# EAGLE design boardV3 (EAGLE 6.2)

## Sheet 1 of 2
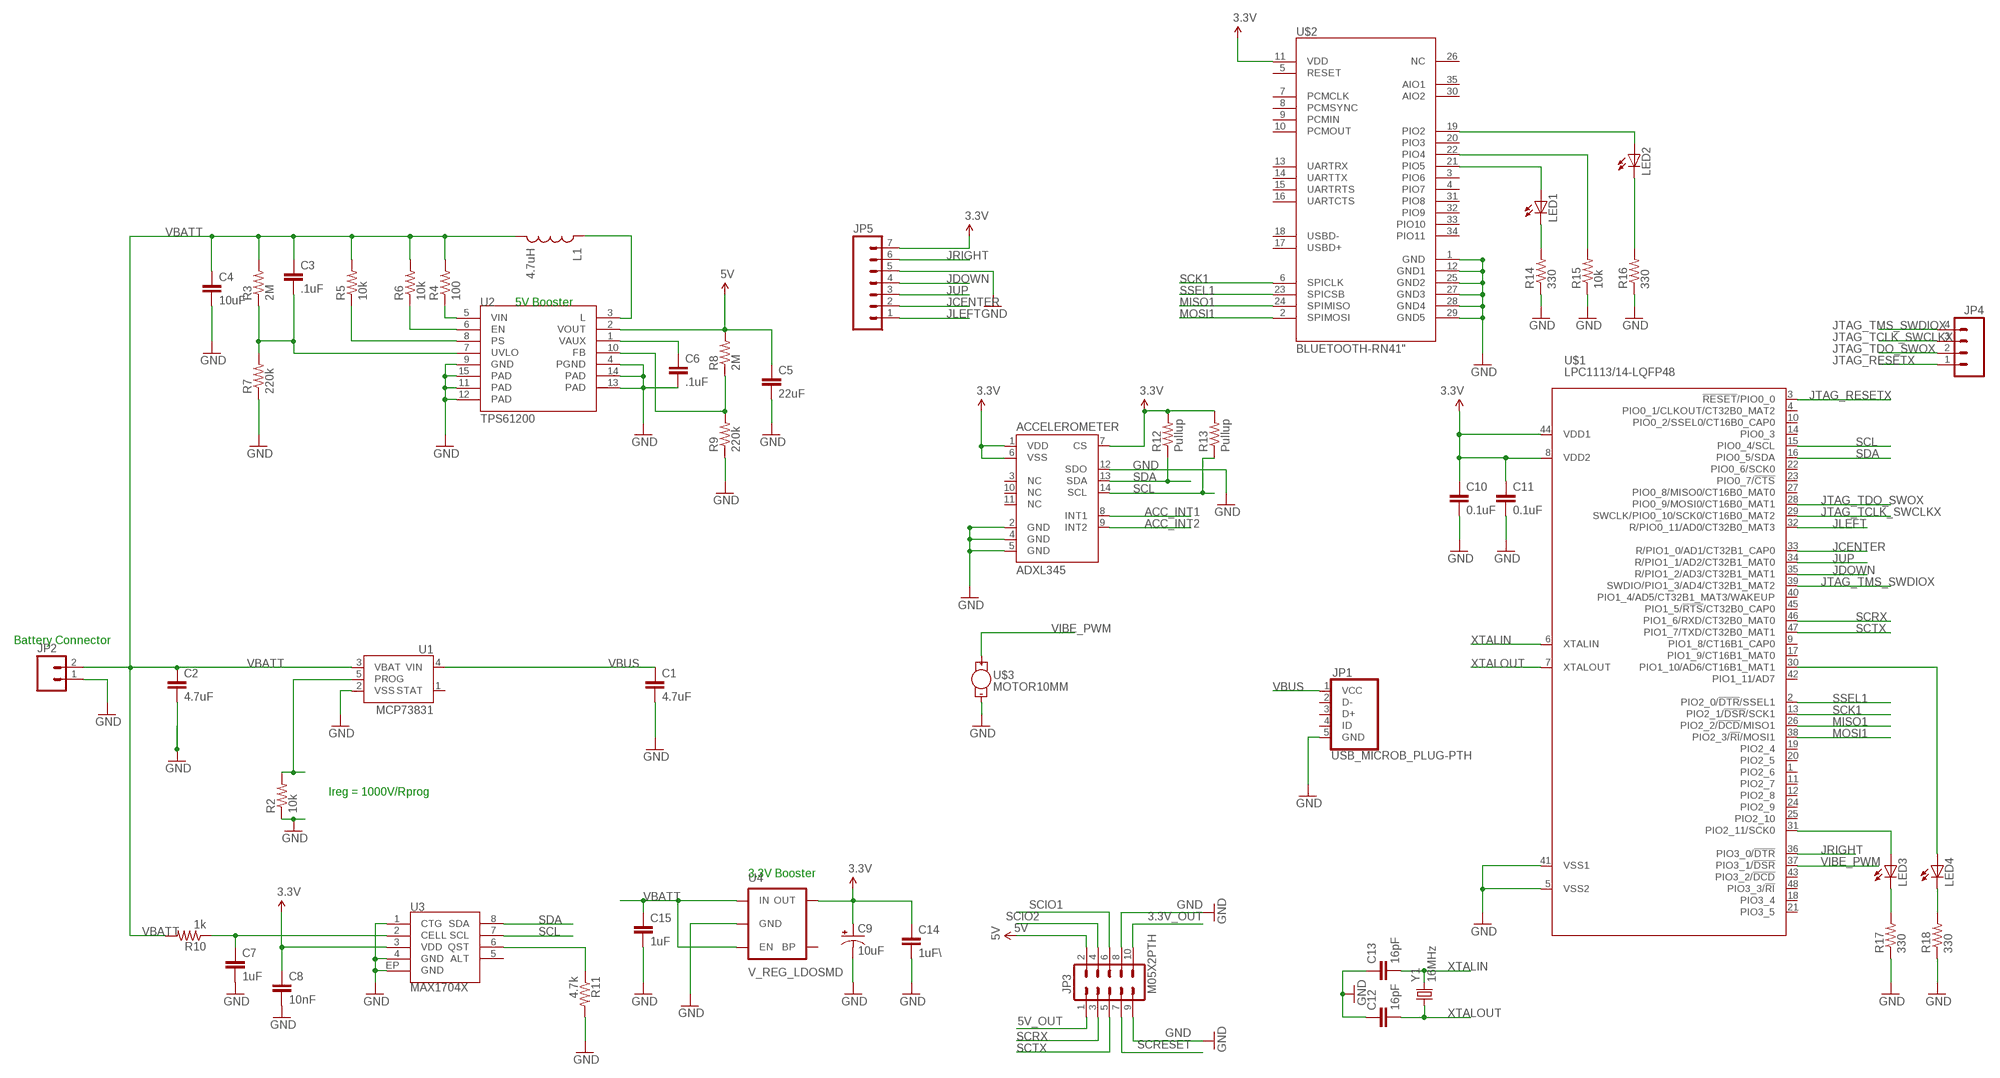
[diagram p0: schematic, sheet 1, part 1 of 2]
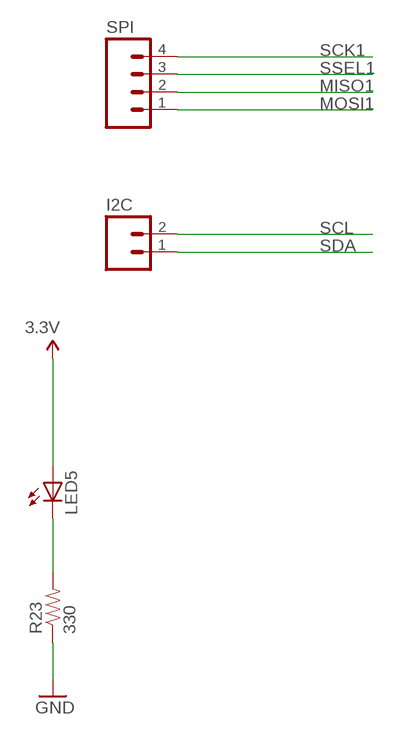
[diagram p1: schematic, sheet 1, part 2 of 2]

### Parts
ACCELEROMETER  ADXL345  [LGA14]
C1  4.7uF  CAP0603-CAP  [0603-CAP]
C2  4.7uF  CAP0603-CAP  [0603-CAP]
C3  .1uF  CAP0603-CAP  [0603-CAP]
C4  10uF  CAP0603-CAP  [0603-CAP]
C5  22uF  CAP0603-CAP  [0603-CAP]
C6  .1uF  CAP0603-CAP  [0603-CAP]
C7  1uF  CAP0603-CAP  [0603-CAP]
C8  10nF  CAP0603-CAP  [0603-CAP]
C9  10uF  10UF-TANT  [EIA3216]
C10  0.1uF  CAP0603-CAP  [0603-CAP]
C11  0.1uF  CAP0603-CAP  [0603-CAP]
C12  16pF  CAP0603-CAP  [0603-CAP]
C13  16pF  CAP0603-CAP  [0603-CAP]
C14  1uF\  CAP0603-CAP  [0603-CAP]
C15  1uF  CAP0603-CAP  [0603-CAP]
I2C  M02POGO_PIN_HOLES_ONLY  [1X02_PP_HOLES_ONLY]
JP1  USB_MICROB_PLUG-PTH  [MICRO-B-RA-TH]
JP2  M02-JST-2-PTH-NO_SILK  [JST-2-PTH-NS]
JP3  M05X2PTH  [AVR_ICSP]
JP4  M04POLAR  [MOLEX-1X4]
JP5  M07  [1X07]
L1  4.7uH  INDUCTOR.  [CDRH2D09]
LED1  LED0603  [LED-0603]
LED2  LED0603  [LED-0603]
LED3  LED0603  [LED-0603]
LED4  LED0603  [LED-0603]
LED5  LED0603  [LED-0603]
R2  10k  RESISTOR0603-RES  [0603-RES]
R3  2M  RESISTOR0603-RES  [0603-RES]
R4  100  RESISTOR0603-RES  [0603-RES]
R5  10k  RESISTOR0603-RES  [0603-RES]
R6  10k  RESISTOR0603-RES  [0603-RES]
R7  220k  RESISTOR0603-RES  [0603-RES]
R8  2M  RESISTOR0603-RES  [0603-RES]
R9  220k  RESISTOR0603-RES  [0603-RES]
R10  1k  RESISTOR0603-RES  [0603-RES]
R11  4.7k  RESISTOR0603-RES  [0603-RES]
R12  Pullup  RESISTOR0402-RES  [0402-RES]
R13  Pullup  RESISTOR0402-RES  [0402-RES]
R14  330  RESISTOR0603-RES  [0603-RES]
R15  10k  RESISTOR0603-RES  [0603-RES]
R16  330  RESISTOR0603-RES  [0603-RES]
R17  330  RESISTOR0603-RES  [0603-RES]
R18  330  RESISTOR0603-RES  [0603-RES]
R23  330  RESISTOR0603-RES  [0603-RES]
SPI  M04POLAR  [MOLEX-1X4]
U1  MCP73831  [SOT23-5]
U2  TPS61200  [QFN-10_PAD]
U3  MAX1704X  [TDFN-8]
U4  V_REG_LDOSMD  [SOT23-5]
U$1  LPC1113/14-LQFP48  [LQFP48]
U$2  BLUETOOTH-RN41"  [RN41]
U$3  MOTOR10MM  [VIBE-MOTOR-10MM]
Y1  16MHz  CRYSTAL5X3  [CRYSTAL-SMD-5X3]

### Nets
3.3V: ACCELEROMETER.1(VDD) ACCELEROMETER.6(VSS) ACCELEROMETER.7(CS) C8.1 C9.A(+) C10.1 C11.1 C14.1 JP5.7 LED5.A R12.2 R13.2 U3.3(VDD) U4.5(OUT) U$1.8(VDD2) U$1.44(VDD1) U$2.11(VDD) ; also sheet 2
3.3V_OUT: JP3.10
5V: C5.1 JP3.2 R8.2 U2.2(VOUT)
5V_OUT: JP3.1
ACC_INT1: ACCELEROMETER.8(INT1)
ACC_INT2: ACCELEROMETER.9(INT2)
GND: ACCELEROMETER.2(GND) ACCELEROMETER.4(GND) ACCELEROMETER.5(GND) ACCELEROMETER.12(SDO) C1.2 C2.2 C4.2 C5.2 C6.2 C7.2 C8.2 C9.C(-) C10.2 C11.2 C12.1 C13.1 C14.2 C15.2 JP1.5(GND) JP2.1 JP3.8 JP3.9 JP5.5 R2.1 R7.1 R9.1 R11.2 R14.1 R15.1 R16.1 R17.1 R18.1 R23.1 U1.2(VSS) U2.4(PGND) U2.9(GND) U2.11(PAD) U2.12(PAD) U2.13(PAD) U2.14(PAD) U2.15(PAD) U3.1(CTG) U3.4(GND) U3.EP(GND) U4.2(GND) U$1.5(VSS2) U$1.41(VSS1) U$2.1(GND) U$2.12(GND1) U$2.25(GND2) U$2.27(GND3) U$2.28(GND4) U$2.29(GND5) U$3.- ; also sheet 2
JCENTER: JP5.2 U$1.33(R/PIO1_0/AD1/CT32B1_CAP0) ; also sheet 2
JDOWN: JP5.4 U$1.35(R/PIO1_2/AD3/CT32B1_MAT1) ; also sheet 2
JLEFT: JP5.1 U$1.32(R/PIO0_11/AD0/CT32B0_MAT3) ; also sheet 2
JRIGHT: JP5.6 U$1.36(PIO3_0/!DTR!) ; also sheet 2
JTAG_RESETX: JP4.1 U$1.3(!RESET!/PIO0_0)
JTAG_TCLK_SWCLKX: JP4.3 U$1.29(SWCLK/PIO0_10/SCK0/CT16B0_MAT2)
JTAG_TDO_SWOX: JP4.2 U$1.28(PIO0_9/MOSI0/CT16B0_MAT1)
JTAG_TMS_SWDIOX: JP4.4 U$1.39(SWDIO/PIO1_3/AD4/CT32B1_MAT2)
JUP: JP5.3 U$1.34(R/PIO1_1/AD2/CT32B1_MAT0) ; also sheet 2
MISO1: SPI.2 U$1.26(PIO2_2/!DCD!/MISO1) U$2.24(SPIMISO)
MOSI1: SPI.1 U$1.38(PIO2_3/!RI!/MOSI1) U$2.2(SPIMOSI)
N$1: LED2.A U$2.19(PIO2)
N$2: R2.2 U1.5(PROG)
N$3: C3.2 R3.1 R7.2 U2.7(UVLO)
N$4: C6.1 U2.1(VAUX)
N$5: R6.1 U2.6(EN)
N$6: R5.1 U2.8(PS)
N$7: L1.P$1 U2.3(L)
N$8: R8.1 R9.2 U2.10(FB)
N$9: C7.1 R10.1 U3.2(CELL)
N$10: R11.1 U3.6(QST)
N$11: R15.2 U$2.22(PIO4)
N$12: LED1.A U$2.21(PIO5)
N$13: LED1.C R14.2
N$14: LED2.C R16.2
N$15: LED3.A U$1.31(PIO2_11/SCK0)
N$16: LED4.A U$1.30(PIO1_10/AD6/CT16B1_MAT1)
N$17: LED3.C R17.2
N$18: LED4.C R18.2
N$21: LED5.C R23.2
SCIO1: JP3.6
SCIO2: JP3.4
SCK1: SPI.4 U$1.13(PIO2_1/!DSR!/SCK1) U$2.6(SPICLK)
SCL: ACCELEROMETER.14(SCL) I2C.2 R13.1 U3.7(SCL) U$1.15(PIO0_4/SCL)
SCRESET: JP3.7
SCRX: JP3.3 U$1.46(PIO1_6/RXD/CT32B0_MAT0)
SCTX: JP3.5 U$1.47(PIO1_7/TXD/CT32B0_MAT1)
SDA: ACCELEROMETER.13(SDA) I2C.1 R12.1 U3.8(SDA) U$1.16(PIO0_5/SDA)
SSEL1: SPI.3 U$1.2(PIO2_0/!DTR!/SSEL1) U$2.23(SPICSB)
VBATT: C2.1 C3.1 C4.1 C15.1 JP2.2 L1.P$2 R3.2 R4.2 R5.2 R6.2 R10.2 U1.3(VBAT) U4.1(IN) U4.3(EN)
VBUS: C1.1 JP1.1(VCC) U1.4(VIN)
VIBE_PWM: U$1.37(PIO3_1/!DSR!) U$3.+
VIN: R4.1 U2.5(VIN)
XTALIN: C13.2 U$1.6(XTALIN) Y1.3
XTALOUT: C12.2 U$1.7(XTALOUT) Y1.1
Unconnected: ACCELEROMETER.3(NC) ACCELEROMETER.10(NC) ACCELEROMETER.11(NC) JP1.2(D-) JP1.3(D+) JP1.4(ID) U1.1(STAT) U3.5(ALT) U4.4(BP) U$1.1(PIO2_6) U$1.4(PIO0_1/CLKOUT/CT32B0_MAT2) U$1.9(PIO1_8/CT16B1_CAP0) U$1.10(PIO0_2/SSEL0/CT16B0_CAP0) U$1.11(PIO2_7) U$1.12(PIO2_8) U$1.14(PIO0_3) U$1.17(PIO1_9/CT16B1_MAT0) U$1.18(PIO3_4) U$1.19(PIO2_4) U$1.20(PIO2_5) U$1.21(PIO3_5) U$1.22(PIO0_6/SCK0) U$1.23(PIO0_7/!CTS!) U$1.24(PIO2_9) U$1.25(PIO2_10) U$1.27(PIO0_8/MISO0/CT16B0_MAT0) U$1.40(PIO1_4/AD5/CT32B1_MAT3/WAKEUP) U$1.42(PIO1_11/AD7) U$1.43(PIO3_2/!DCD!) U$1.45(PIO1_5/!RTS!/CT32B0_CAP0) U$1.48(PIO3_3/!RI!) U$2.3(PIO6) U$2.4(PIO7) U$2.5(RESET) U$2.7(PCMCLK) U$2.8(PCMSYNC) U$2.9(PCMIN) U$2.10(PCMOUT) U$2.13(UARTRX) U$2.14(UARTTX) U$2.15(UARTRTS) U$2.16(UARTCTS) U$2.17(USBD+) U$2.18(USBD-) U$2.20(PIO3) U$2.26(NC) U$2.30(AIO2) U$2.31(PIO8) U$2.32(PIO9) U$2.33(PIO10) U$2.34(PIO11) U$2.35(AIO1)

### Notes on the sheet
- 5V Booster
- Battery Connector
- Ireg = 1000V/Rprog
- 3.3V Booster

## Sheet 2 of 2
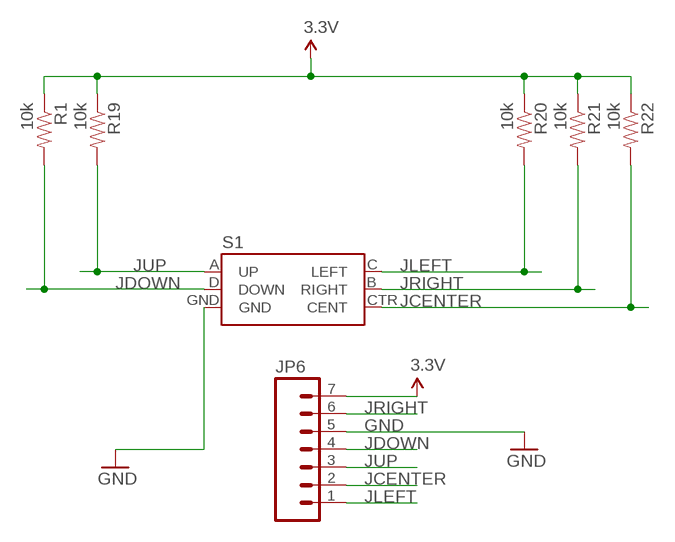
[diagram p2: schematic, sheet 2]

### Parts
JP6  M07  [1X07]
R1  10k  RESISTOR0603-RES  [0603-RES]
R19  10k  RESISTOR0603-RES  [0603-RES]
R20  10k  RESISTOR0603-RES  [0603-RES]
R21  10k  RESISTOR0603-RES  [0603-RES]
R22  10k  RESISTOR0603-RES  [0603-RES]
S1  JOYSTICK_MINI  [JOYSTICK_MINI]

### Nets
3.3V: JP6.7 R1.1 R19.1 R20.1 R21.1 R22.1 ; also sheet 1
GND: JP6.5 S1.GND ; also sheet 1
JCENTER: JP6.2 R22.2 S1.CTR(CENT) ; also sheet 1
JDOWN: JP6.4 R1.2 S1.D(DOWN) ; also sheet 1
JLEFT: JP6.1 R20.2 S1.C(LEFT) ; also sheet 1
JRIGHT: JP6.6 R21.2 S1.B(RIGHT) ; also sheet 1
JUP: JP6.3 R19.2 S1.A(UP) ; also sheet 1

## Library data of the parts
ACCELEROMETER = SparkFun-Sensors:ADXL345: 3-axis SPI/I2C 2/4/8/16g accelerometer
C1-C8 C10-C15 = SparkFun-Passives:CAP: Capacitor
C9 = SparkFun-Capacitors:10UF-TANT: 10uF Tantalum SMT; PROD_ID: CAP-00811
I2C JP2 = SparkFun-Connectors:M02: Header 2
JP1 = SparkFun-Connectors:USB_MICROB_PLUG: USB Micro-B Plug Comes in a variety of packages. Check out Hirose's ZX-x0 line: http://www.hirose.co.jp/cataloge_hp/e24200011.pdf
JP3 = SparkFun-Connectors:M05X2: Header 5x2 Standard 10-pin dual row 0.1" header. Commonly used with AVR-ISP. Use with Spark Fun Electronics SKU: PRT-00778
JP4 SPI = SparkFun-Connectors:M04: Header 4 Standard 4-pin 0.1" header. Use with straight break away headers (SKU : PRT-00116), right angle break away headers (PRT-00553), swiss pins (PRT-00743), machine pins (PRT-00117), and female headers (PRT-00115). Molex polarized connector foot print use with SKU : PRT-08231 with associated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
JP5 JP6 = SparkFun-Connectors:M07: Header 7 Standard 7-pin 0.1" header. Use with straight break away headers (SKU : PRT-00116), right angle break away headers (PRT-00553), swiss pins (PRT-00743), machine pins (PRT-00117), and female headers (PRT-00115). NOTES ON THE VARIANTS LOCK and LOCK_LONGPADS... This footprint was designed to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
L1 = SparkFun-Passives:INDUCTOR: Inductors
LED1-LED5 = SparkFun-LED:LED: LEDs
R1 R8 R9 R19-R22 = SparkFun-Resistors:RESISTOR: Resistor
R2-R7 R10-R18 R23 = SparkFun-Passives:RESISTOR: Resistor
S1 = SparkFun-Electromechanical:JOYSTICK_MINI: Small 5-way tactile joystick, COM-10063 4UCON SF303GJ26
U1 = SparkFun-PowerIC:MCP73831: Miniature single cell, fully integrated Li-Ion, Li-polymer charge management controller http://ww1.microchip.com/downloads/en/DeviceDoc/21984a.pdf IC-09995; PROD_ID: IC-09995
U2 = SparkFun-PowerIC:TPS61200: DC to DC Booster IC-10035; PROD_ID: IC-10035
U3 = SparkFun-PowerIC:MAX1704X: MAX17043/MAX17044: Battery Fuel Guage (43 is 1cell, 44 is 2cell)
U4 = SparkFun-PowerIC:V_REG_LDO: Voltage Regulator LDO Standard 150mA LDO voltage regulator in SOT-23 layout. Micrel part MIC5205. BP (by-pass) pin is used to lower output noise with 470pF cap.
U$1 = lpc1100v1.1:LPC1113/14-LQFP48: NXP Semiconductors LPC11xx microcontrollers ARM 32-bit Cortex-M0 Microcontroller with MPU CPU clock up to 50MHz Up to 32KByte on-chip Flash ROM with In-System Programming (ISP) and In-Application Programming (IAP) via On-Chip Bootloader Up to 8KByte SRAM Nested Vectored Interrupt Controller Up to 2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
U$2 = SparkFun-RF:BLUETOOTH-RN41: Bluetooth SMD module
U$3 = SparkFun-Electromechanical:MOTOR: Vibration Motor- ROB-08449
Y1 = SparkFun-FreqCtrl:CRYSTAL: Various standard crystals. Proven footprints. Spark Fun Electronics SKU : COM-00534

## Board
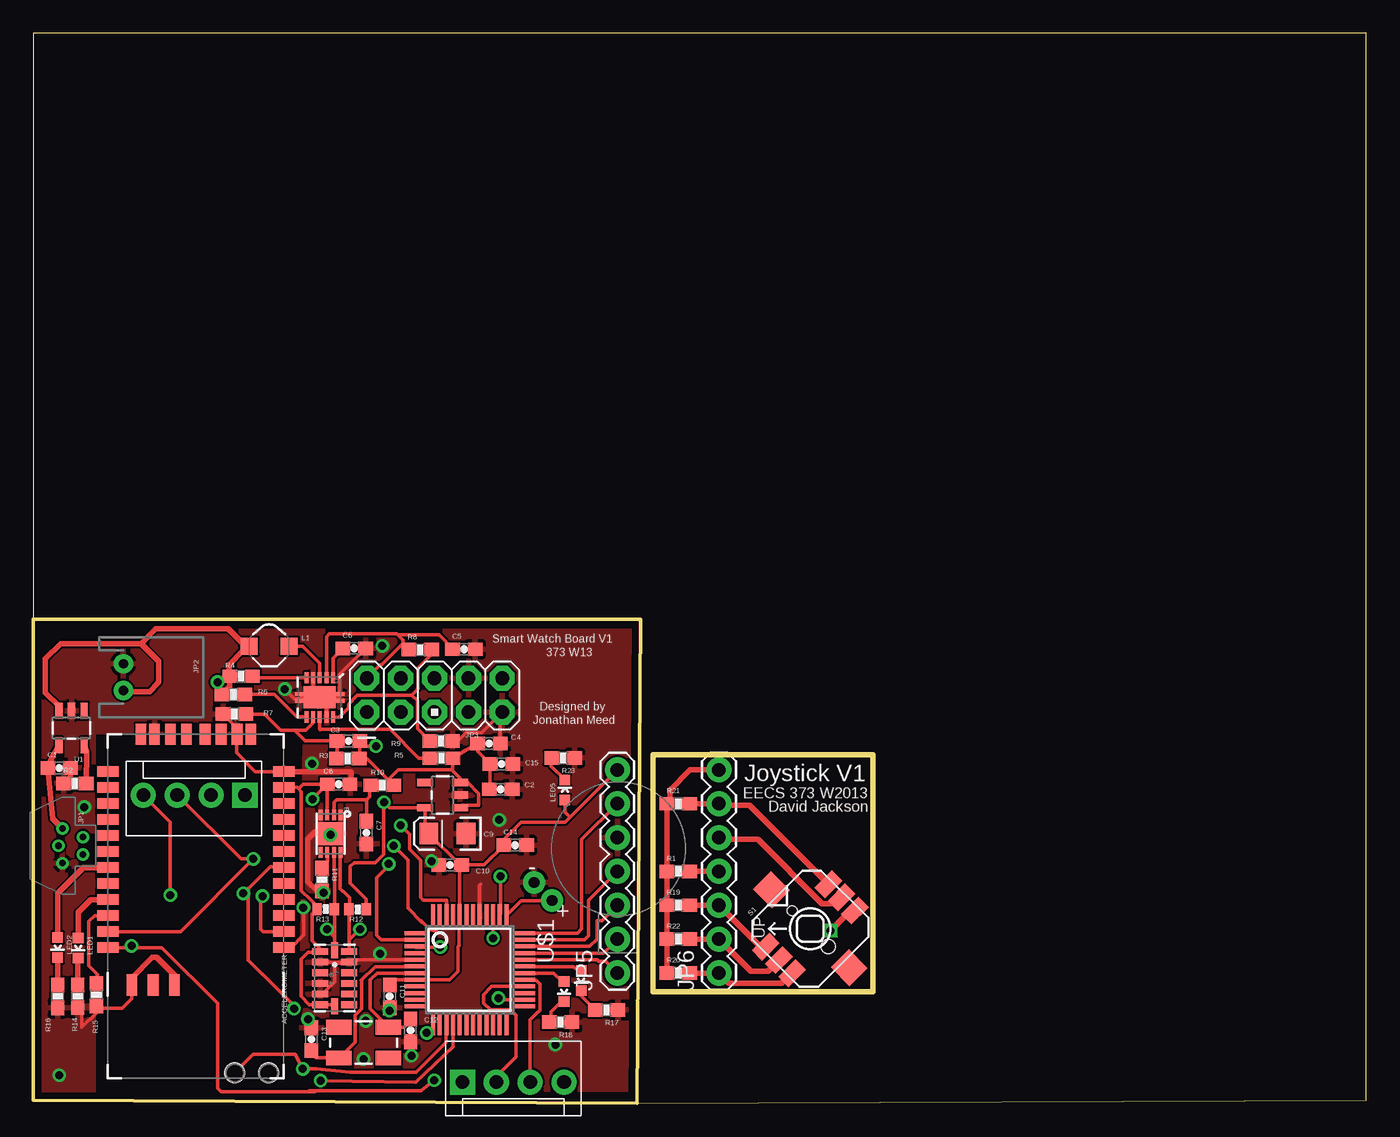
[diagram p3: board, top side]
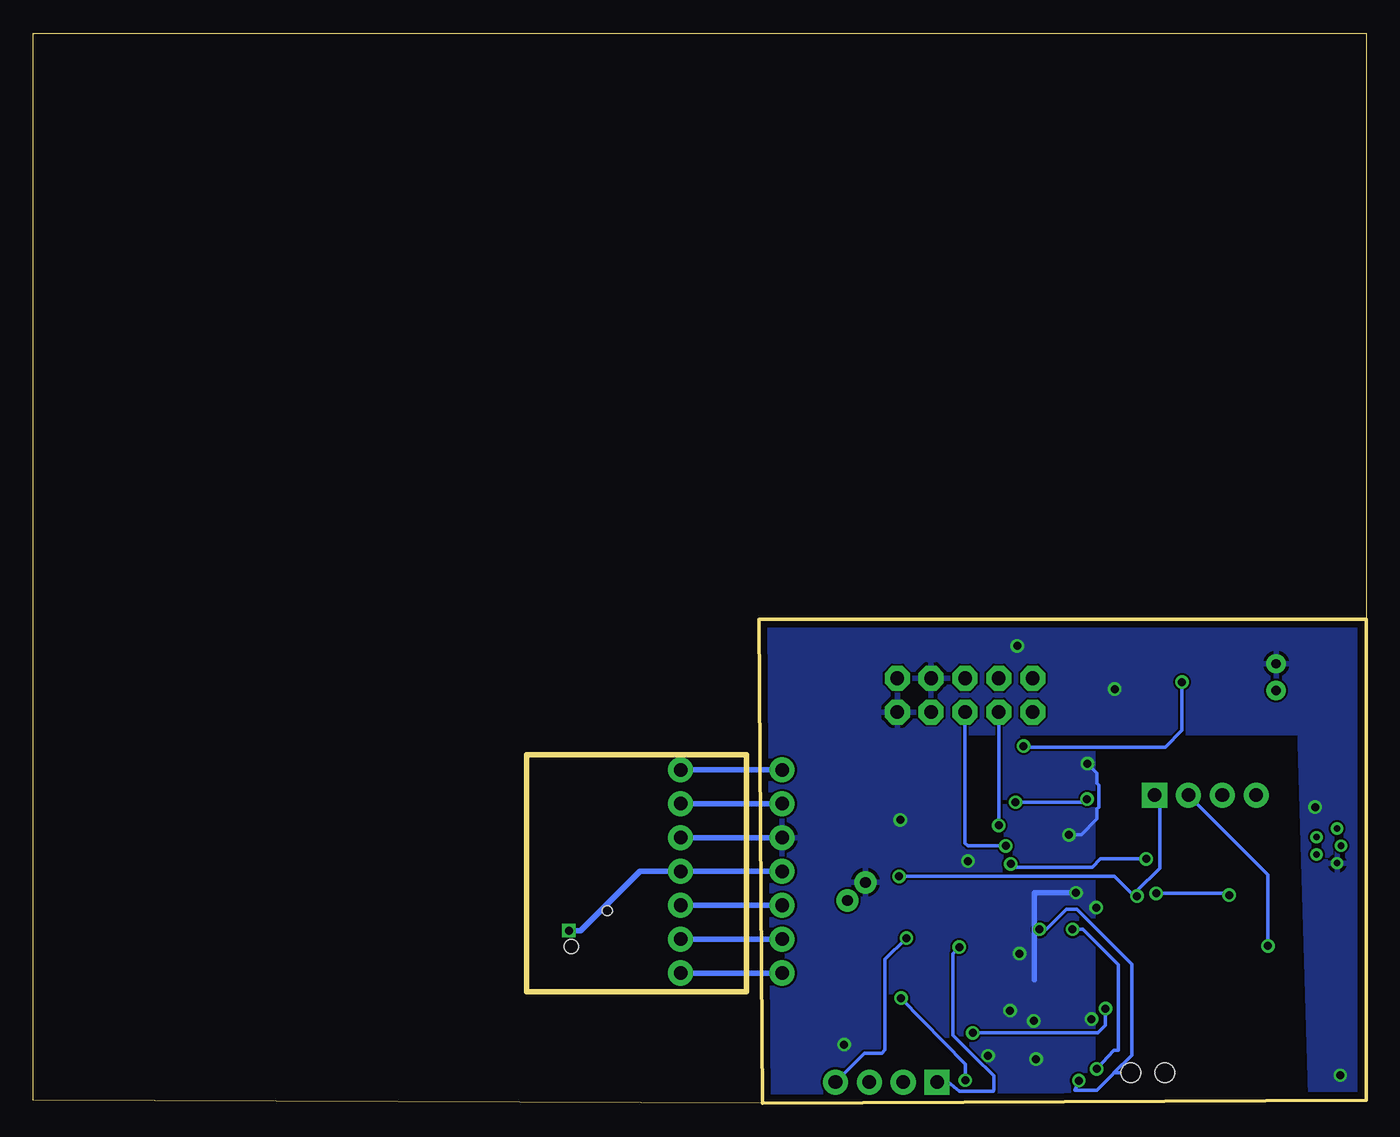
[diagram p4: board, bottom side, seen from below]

Size 100 x 80.25 mm. Coordinates in mm from the lower left corner, seen from the top.
Outline: 45.31,0 100,0.25 100,80.25 0,80.25 0,36.33
Outline: 0,36.33 0,0.25 45.31,0
Outline: 45.31,0 45.56,36.33 0,36.33
Outline: 46.48,8.38 46.48,26.16 62.99,26.16 62.99,8.38 46.48,8.38
Copper layers (1*16): Top 0.0178mm / dielectric 59mil / Bottom 0.0178mm
Design rules: minimum track width 6mil, minimum drill 14mil, track to track 6mil, track to pad 6mil, pad to pad 6mil, via to via 6mil, smd to smd 6mil, copper to edge 20mil, drill to drill 16mil, minimum pad ring 8mil, minimum via ring 8mil, stop-mask expansion 3mil, vias tented up to drill 0mil, thermal gap 10mil

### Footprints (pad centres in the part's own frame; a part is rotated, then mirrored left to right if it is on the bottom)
LGA14 = smd 0.5 x 1.2: 1 2,1.1; 2 1.2,1.1; 3 0.4,1.1; 4 -0.4,1.1; 5 -1.2,1.1; 6 -2,1.1; 8 -2,-1.1; 9 -1.2,-1.1; 10 -0.4,-1.1; 11 0.4,-1.1; 12 1.2,-1.1; 13 2,-1.1 | smd 1.2 x 0.5: 7 -2.1,0; 14 2.1,0
0603-CAP = smd 1.1 x 1: 1 -0.85,0; 2 0.85,0
EIA3216 = smd 1.4 x 1.6: A 1.4,0; C -1.4,0
1X02_PP_HOLES_ONLY = drill 0.889 pad 0.813: 1 0,0; 2 2.54,0 | hole 1.473: 0,0; 2.54,0
MICRO-B-RA-TH = drill 0.508 pad 0.9: 1 -1.3,-0.95; 2 -0.65,0.6; 3 0,-1.25; 4 0.65,0.6; 5 1.3,-0.95
JST-2-PTH-NS = drill 0.7 pad 1.448: 1 -1,0; 2 1,0
AVR_ICSP = drill 1.016 pad 1.88 octagon: 1 -1.27,5.08; 2 1.27,5.08; 3 -1.27,2.54; 4 1.27,2.54; 5 -1.27,0; 6 1.27,0; 7 -1.27,-2.54; 8 1.27,-2.54; 9 -1.27,-5.08; 10 1.27,-5.08
MOLEX-1X4 = drill 1.016 pad 1.88 square: 1 0,0 | drill 1.016 pad 1.88: 2 2.54,0; 3 5.08,0; 4 7.62,0
1X07 = drill 1.016 pad 1.88: 1 0,0; 2 2.54,0; 3 5.08,0; 4 7.62,0; 5 10.16,0; 6 12.7,0; 7 15.24,0
CDRH2D09 = smd 1.3 x 1.3: P$1 -1.5,0; P$2 1.5,0
LED-0603 = smd 0.8 x 0.8: A 0,-0.75; C 0,0.75
0603-RES = smd 1.1 x 1: 1 -0.85,0; 2 0.85,0
0402-RES = smd 0.7 x 0.9: 1 -0.65,0; 2 0.65,0
JOYSTICK_MINI = smd 1.85 x 1.1: A -3.325,1.4; B 3.325,1.4; C -3.325,-1.4; CTR -3.325,0; D 3.325,-1.4; GND 3.325,0 | smd 1.9 x 2: NC 0,4.13; NC@0 0,-4.13 | hole 0.75: 0,1.9 | hole 1.05: 0,-1.9
SOT23-5 = smd 0.55 x 1.2: 1 -0.95,-1.3; 2 0,-1.3; 3 0.95,-1.3; 4 0.95,1.3; 5 -0.95,1.3
QFN-10_PAD = smd 0.297 x 0.85: 1 -1,-1.475; 2 -0.5,-1.475; 3 0,-1.475; 4 0.5,-1.475; 5 1,-1.475; 6 1,1.475; 7 0.5,1.475; 8 0,1.475; 9 -0.5,1.475; 10 -1,1.475 | smd 0.7 x 0.28: 11 -1.5,0.25; 12 -1.5,-0.25; 13 1.5,0.25; 14 1.5,-0.25 | smd 2.4 x 1.65: 15 0,0
TDFN-8 = smd 0.8 x 0.3: 1 -1.4,0.75; 2 -1.4,0.25; 3 -1.4,-0.25; 4 -1.4,-0.75; 5 1.4,-0.75; 6 1.4,-0.25; 7 1.4,0.25; 8 1.4,0.75 | smd 1.73 x 1.88: EP 0,0
LQFP48 = smd 0.3 x 1.6: 1 -2.75,-4.1; 2 -2.25,-4.1; 3 -1.75,-4.1; 4 -1.25,-4.1; 5 -0.75,-4.1; 6 -0.25,-4.1; 7 0.25,-4.1; 8 0.75,-4.1; 9 1.25,-4.1; 10 1.75,-4.1; 11 2.25,-4.1; 12 2.75,-4.1; 25 2.75,4.1; 26 2.25,4.1; 27 1.75,4.1; 28 1.25,4.1; 29 0.75,4.1; 30 0.25,4.1; 31 -0.25,4.1; 32 -0.75,4.1; 33 -1.25,4.1; 34 -1.75,4.1; 35 -2.25,4.1; 36 -2.75,4.1 | smd 1.6 x 0.3: 13 4.1,-2.75; 14 4.1,-2.25; 15 4.1,-1.75; 16 4.1,-1.25; 17 4.1,-0.75; 18 4.1,-0.25; 19 4.1,0.25; 20 4.1,0.75; 21 4.1,1.25; 22 4.1,1.75; 23 4.1,2.25; 24 4.1,2.75; 37 -4.1,2.75; 38 -4.1,2.25; 39 -4.1,1.75; 40 -4.1,1.25; 41 -4.1,0.75; 42 -4.1,0.25; 43 -4.1,-0.25; 44 -4.1,-0.75; 45 -4.1,-1.25; 46 -4.1,-1.75; 47 -4.1,-2.25; 48 -4.1,-2.75
RN41 = smd 0.8 x 1.6: 1 -6.6,-6.6; 2 -5.4,-6.6; 3 -4.2,-6.6; 4 -3,-6.6; 5 -1.8,-6.6; 6 -0.6,-6.6; 7 0.6,-6.6; 8 1.8,-6.6; 9 3,-6.6; 10 4.2,-6.6; 11 5.4,-6.6; 12 6.6,-6.6; 13 6.6,6.6; 14 5.4,6.6; 15 4.2,6.6; 16 3,6.6; 17 1.8,6.6; 18 0.6,6.6; 19 -0.6,6.6; 20 -1.8,6.6; 21 -3,6.6; 22 -4.2,6.6; 23 -5.4,6.6; 24 -6.6,6.6 | smd 1.6 x 0.8: 25 -9.4,4.8; 26 -9.4,3.2; 27 -9.4,1.6; 28 9.4,3.1; 29 9.4,-3.1; 30 9.4,-4.122; 31 9.4,-1.9; 32 9.4,-0.7; 33 9.4,0.7; 34 9.4,1.9; 35 9.4,4.122
VIBE-MOTOR-10MM = drill 0.8 pad 1.676: + -5,-3.9; - -6.35,-2.54
CRYSTAL-SMD-5X3 = smd 1.9 x 1.1: 1 -1.85,-1.15; 2 1.85,-1.15; 3 1.85,1.15; 4 -1.85,1.15

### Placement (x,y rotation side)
ACCELEROMETER  22.61,9.4 90 top
C1  1.95,25.16 0 top
C2  35.07,23.56 0 top
C3  23.64,27.18 180 top
C4  34.18,26.99 0 top
C5  32.31,34.06 0 top
C6  24.09,34.12 0 top
C7  24.98,20.32 270 top
C8  22.9,23.94 0 top
C9  31.07,20.24 180 top
C10  31.28,17.88 180 top
C11  26.74,8.02 270 top
C12  28.3,5.47 90 top
C13  20.87,4.82 270 top
C14  36.16,19.37 0 top
C15  35.12,25.46 0 top
I2C  17.65,2.29 180 top
JP1  3.13,19.32 270 top
JP2  6.75,31.97 270 top
JP3  30.1,30.61 90 top
JP4  32.2,1.6 0 top
JP5  43.81,9.78 90 top
JP6  51.44,9.78 90 top
L1  17.69,34.28 180 top
LED1  3.36,11.66 180 top
LED2  1.82,11.69 180 top
LED3  41.1,9.22 180 top
LED4  39.82,8.39 180 top
LED5  39.88,23.5 0 top
R1  48.39,17.4 0 top
R2  3.12,23.99 0 top
R3  23.59,25.87 0 top
R4  15.59,32.03 180 top
R5  30.62,25.89 0 top
R6  15.01,30.67 180 top
R7  15.09,29.2 0 top
R8  29.03,34.03 180 top
R9  30.59,27.18 180 top
R10  26.19,23.85 0 top
R11  21.66,16.78 270 top
R12  24.34,14.55 0 top
R13  21.94,14.58 180 top
R14  3.33,8.04 90 top
R15  4.74,8.15 90 top
R16  1.83,8.03 90 top
R17  43,7.01 180 top
R18  39.55,6.09 180 top
R19  48.39,14.86 0 top
R20  48.39,9.78 0 top
R21  48.39,22.48 0 top
R22  48.39,12.32 0 top
R23  39.75,25.91 180 top
S1  58.29,13.1 45 top
SPI  15.88,23.11 180 top
U1  2.86,28.16 180 top
U2  21.49,30.45 180 top
U3  22.31,20.24 270 top
U4  30.71,23.13 90 top
U$1  32.74,10.02 270 top
U$2  12.19,18.29 90 top
U$3  43.92,19.11 0 top
Y1  24.78,4.56 180 top

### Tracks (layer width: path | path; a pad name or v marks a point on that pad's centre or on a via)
3.3V  (via drill 0.6)
  Top 0.254: ACCELEROMETER.7 22.51,7.4 ACCELEROMETER.6 20.7,7.4 20.08,8.03 20.08,10.79 20.61,11.32 21.43,11.32 ACCELEROMETER.1 | ACCELEROMETER.1 21.51,11.31 21.55,11.27 | ACCELEROMETER.1 21.51,11.6 20.92,12.19 20.92,14.21 R13.2 21.29,14.77 20.79,15.27 | 20.79,15.27 | 20.79,15.27 20.11,15.96 20.11,23.39 19.89,23.6 | 19.89,23.6 19.79,23.7 18.81,23.7 U$2.11 | C8.1 U3.3 | C8.1 20.23,23.94 19.89,23.6 | v20.95,22.82 v20.95,22.83 C8.1 | C9.A 29.41,20.49 U4.5 26.72,22.18 v26.31,22.59 26.27,22.55 26.27,18.68 25.64,18.05 24.06,18.05 23.79,17.77 23.79,16.51 24.98,15.31 R12.2 | 30,19.91 C9.A | C10.1 32.2,17.88 | 32.2,17.88 | C10.1 32.02,17.88 C9.A | C11.1 27.13,9.27 U$1.8 31.24,9.27 31.88,9.91 31.88,11.75 31.95,11.82 31.95,14.08 U$1.44 31.99,17.74 C10.1 | 32.2,17.88 33.82,17.88 C14.1 35.31,19.81 36.58,21.08 39.88,21.08 40.26,21.46 | 40.26,21.46 JP5.7 | LED5.A 39.88,21.84 40.26,21.46
  Top 0.406: JP6.7 49.28,25.02 47.75,23.5 47.75,22.69 R21.1 R1.1 R19.1 R22.1 R20.1
  Bottom 0.254: v26.31,22.59 21.18,22.59 v20.95,22.82
  Bottom 0.406: JP5.7 JP6.7
5V
  Top 0.254: U2.2 21.99,35.01 22.2,35.22 27.27,35.22 27.38,35.1 | 27.38,35.1 27.75,34.74 27.75,34.52 27.59,34.37 | 27.59,34.37 26.12,32.89 26.03,32.89 JP3.2 | R8.2 27.93,34.03 27.59,34.37 | C5.1 31.46,34.12 30.44,35.13 27.41,35.13 27.38,35.1
GND  (via drill 0.6)
  Top 0.254: ACCELEROMETER.5 21.67,8.2 22.61,9.13 22.61,10.4 22.71,10.5 23.61,10.5 ACCELEROMETER.12 | ACCELEROMETER.12 ACCELEROMETER.2 | 18.79,25.26 U$2.12 16.64,24.89 15.24,26.29 15.24,27.64 U$2.29 15.53,27.93 15.51,27.93 R7.1 | U$1.5 23.88,10.77 ACCELEROMETER.12 | U$2.25 7.39,7.84 6.67,7.13 4.92,7.13 R15.1 4.74,6.8 3.65,5.7 3.65,6.87 R14.1 | U$2.1 19.34,11.69 20.29,12.64 20.29,14.64 v20.25,14.68 | 33.49,14 U$1.41 33.49,16.37 33.54,16.42 | 33.49,14 33.51,13.99 | 33.49,14 33.49,13.95 33.55,13.89 | U2.12 22.99,32.18 C6.2 | C4.2 35.03,29.2 JP3.9 33.65,27.81 32.48,27.81 31.84,27.18 R9.1 | U2.4 20.99,30.95 | U2.9 21.99,30.21 21.84,30.35 19.56,30.35 18.92,30.99 18.8,30.99 | C11.2 26.74,6.98 v26.72,6.95
  Top 0.406: U$2.25 7.39,9.4 8.94,10.94 9.26,10.94 10.63,9.57 10.63,8.93 U$2.27 | 3.44,7.28 R14.1 | C1.2 2.75,24.03 R2.1 | U$2.12 23.82,24.89 23.83,24.88 23.83,24.01 C8.2 | 20.99,30.95 U2.15 | U2.15 20.24,30.45 U2.13 | U2.15 22.74,30.45 U2.12 | JP6.5 51.44,19.81 54.36,19.81 59.18,14.99 60.18,14.99 S1.GND | R11.2 21.28,15.93 20.57,16.64 20.57,19.81 21.14,20.38 22.16,20.38 U3.EP
  Bottom 0.254: v22.3,20.14 21.39,20.14 20.19,21.34 20.19,22.1 20.07,22.23 20.07,23.88 20.19,24 20.19,24.77 v20.9,25.48
  Bottom 0.406: JP5.5 JP6.5 | v21.77,15.8 24.89,15.8 24.89,9.27
  other vias: 1.94,2.11 3.83,22.23 28.38,3.57 20.61,6.31 24.77,3.33 24.94,6.19 26.01,11.23 26.18,34.31 29.88,18.17 34.96,21.26 18.87,31.06 39.16,4.41
  pour Bottom: 4.94,35.71 45.05,35.71 45.05,27.81 4.94,27.81 4.94,33.06
  pour Top: 4.81,35.46 45.03,35.46 45.03,27.86 4.58,27.86
  pour Top: 0.45,35.55 4.49,35.55 4.49,0.66 0.58,0.66 0.58,1.6
  pour Top: 20.4,27.59 45.21,27.59 45.21,1.06 20.09,1.06 20.09,2.73
  pour Bottom: 0.47,35.86 5.19,35.86 4.16,0.57 0.62,0.57 0.62,0.77
  pour Bottom: 20.58,27.55 45.36,27.55 45.36,0.57 21.61,0.57 21.61,0.83 20.52,0.83 20.52,27.49
JCENTER
  Top 0.254: U$1.33 42.76,11.27 JP5.2
  Top 0.406: R22.2 JP6.2 53.85,9.91 55.12,9.91 55.94,10.73 S1.CTR
  Bottom 0.406: JP5.2 JP6.2
JDOWN  (via drill 0.6)
  Top 0.254: U$1.35 41.35,12.27 41.66,12.57 41.66,15.24 JP5.4
  Top 0.406: S1.D 61.61,14.46 61.59,14.48 61.34,14.48 v59.82,12.95 | JP6.4 R1.2
  Bottom 0.406: v59.82,12.95 58.93,12.95 54.48,17.4 JP6.4 JP5.4
JLEFT
  Top 0.254: U$1.32 42.32,10.77 42.42,10.67 42.93,10.67 JP5.1
  Top 0.406: R20.2 JP6.1 52.2,9.02 56.13,9.02 56.88,9.76 S1.C
  Bottom 0.406: JP5.1 JP6.1
JRIGHT
  Top 0.254: U$1.36 40.84,12.77 41.15,13.08 41.15,19.81 JP5.6
  Top 0.406: R21.2 JP6.6 51.56,22.35 53.74,22.35 S1.B
  Bottom 0.406: JP5.6 JP6.6
JTAG_RESETX  (via drill 0.6)
  Top 0.254: v30.53,11.72 28.68,11.72 U$1.3
  Bottom 0.254: JP4.1 31.35,1.6 30.51,0.89 27.97,0.89 27.91,1.09 27.91,2.07 28.57,2.73 28.75,2.85 31.02,5.12 31.02,11.23 v30.53,11.72
JTAG_TCLK_SWCLKX
  Top 0.254: JP4.3 37.28,6.27 37.88,6.87 37.91,6.87 38.03,6.99 38.03,8.94 37.73,9.25 36.86,9.25 U$1.29
JTAG_TDO_SWOX
  Top 0.254: U$1.28 34.4,8.77 33.79,8.17 33.79,7.53 34.3,7.02 35.81,7.02 36.23,6.6 36.23,3.52 34.86,2.14 34.86,1.73 JP4.2
JTAG_TMS_SWDIOX  (via drill 0.6)
  Top 0.254: v34.49,12.4 U$1.39
  Bottom 0.254: JP4.4 | JP4.4 37.65,3.77 36.34,3.77 36.09,4.01 36.09,10.79 v34.49,12.4
JUP
  Top 0.254: U$1.34 41.74,11.77 42.29,12.32 42.29,13.72 42.67,13.72 JP5.3
  Top 0.406: R19.2 JP6.3 54.56,11.74 S1.A
  Bottom 0.406: JP5.3 JP6.3
MISO1  (via drill 0.6)
  Top 0.254: 20.77,0.95 20.7,0.95 | 20.7,0.95 29.09,0.93 v30.07,1.74 | U$1.26 35.03,7.77 v34.9,7.9 | U$2.24 7.49,11.69 | 20.7,0.95 21.15,0.89 14.1,0.89 13.84,1.14 13.84,7.49 9.65,11.69 7.49,11.69 | 7.49,11.69 v7.37,11.81
  Bottom 0.254: v30.07,1.74 30.07,2.94 v34.9,7.9 | v7.37,11.81 7.37,17.14 SPI.2
MOSI1  (via drill 0.6)
  Top 0.254: U$2.2 17.23,12.89 17.04,13.07 17.04,15.39 v17.19,15.54 | v35.05,17.03 35.05,14.17 U$1.38
  Bottom 0.254: v35.05,17.03 35.04,17.02 18.89,17.02 17.41,15.54 v17.19,15.54 17.19,15.95 15.49,17.65 15.49,22.73 SPI.1
N$1
  Top 0.406: LED2.A 1.82,15.75 3.76,17.68 U$2.19
N$2
  Top 0.406: R2.2 3.99,26.37 U1.5
N$3
  Top 0.254: R7.2 17.35,29.2 18.57,27.97 19.6,27.97 | R3.1 22.79,25.92 C3.2 20.39,27.18 19.6,27.97 | U2.7 20.99,28.54 20.42,27.97 19.6,27.97
N$4
  Top 0.254: U2.1 22.49,33.38 C6.1
N$5
  Top 0.254: R6.1 18.07,30.67 19.22,29.52 19.25,29.52 19.76,29.01 20.46,29.01 U2.6
N$6
  Top 0.254: U2.8 21.49,28.08 21.54,28.04 21.56,28.06 26.75,28.06 28.92,25.89 R5.1
N$7
  Top 0.254: L1.P$1 20.2,34.28 21.46,33.02 21.46,31.95 U2.3
N$8
  Top 0.254: U2.10 22.96,28.97 23.64,29.65 23.64,29.95 24.31,30.62 28.39,30.62 | 28.39,30.62 28.81,30.2 28.81,28.1 R9.2 | 28.39,30.62 28.88,31.11 28.88,32.68 29.88,33.69 R8.1
N$9
  Top 0.254: U3.2 22.55,22.58 22.75,22.78 24.93,22.78 | 24.93,22.78 25.02,22.68 25.02,21.21 C7.1 | 24.93,22.78 25,22.78 25.23,22.99 25.23,23.84 R10.1
N$10
  Top 0.254: R11.1 21.79,17.9 22.08,18.2 22.08,18.81 U3.6
N$11
  Top 0.254: U$2.22 4.59,14.09 4.15,13.65 4.15,10.31 4.83,9.63 4.74,9.54 R15.2
N$12
  Top 0.406: LED1.A 3.36,14.33 4.3,15.26 5.56,15.26 U$2.21
N$13
  Top 0.406: R14.2 3.33,10.88 LED1.C
N$14
  Top 0.406: R16.2 LED2.C
N$15
  Top 0.254: LED3.A 40.82,9.97 40.53,10.27 U$1.31
N$16
  Top 0.254: LED4.A 39.65,9.14 39.04,9.76 U$1.30
N$17
  Top 0.254: LED3.C 41.1,8.06 R17.2
N$18
  Top 0.254: LED4.C 39.62,7.64 38.84,6.86 38.84,6.23 R18.2
N$21
  Top 0.254: LED5.C 39.88,24.26 38.86,25.27 38.86,25.87 R23.2
SCK1  (via drill 0.6)
  Top 0.254: U$1.13 29.99,5.77 v29.51,5.29 | v19.55,7.1 19.55,7.34 17.15,9.74 17.13,9.74 16.13,10.74 16.13,16.1 | U$2.6 18.73,17.75 17.79,17.75 16.13,16.1 | 16.13,16.1 16.1,16.1 v15.75,15.75 | v10.29,15.62 10.29,21.08 SPI.4
  Bottom 0.254: v29.51,5.29 20.13,5.29 19.55,5.87 v19.55,7.1 | v15.75,15.75 10.41,15.75 v10.29,15.62
SCL  (via drill 0.6)
  Top 0.254: U3.7 22.59,15.91 R13.1 22.61,14.56 ACCELEROMETER.14 22.61,12.48 v22.03,13.06 | U$1.15 30.96,5.89 30.96,4.57 28.72,2.33 23.77,2.33 21.23,2.59 v20.22,2.59 19.64,3.68 16.51,3.68 I2C.2
  Bottom 0.254: v22.03,13.06 21.26,13.06 18.6,10.4 18.6,4 18.95,4 v20.22,2.59
SCRX  (via drill 0.6)
  Top 0.254: U$1.46 30.99,15.24 30.99,15.25 29.26,15.25 29.05,15.46 29.05,18.25 28.23,19.06 28.23,20.18 v27.56,20.85
  Bottom 0.254: v27.56,20.85 JP3.3
SCTX  (via drill 0.6)
  Top 0.254: U$1.47 30.49,13.22 30.16,12.89 29.8,13.02 29.11,13.71 29.15,13.59 28.12,14.62 28.12,18.24 v27.05,19.31
  Bottom 0.254: v27.05,19.31 29.9,19.31 30.11,19.52 JP3.5
SDA  (via drill 0.6)
  Top 0.254: v24.5,13.06 23.71,12.26 ACCELEROMETER.13 23.68,11.42 R12.1 23.71,14.58 23.71,15.43 23.23,15.91 23.2,15.91 23.03,16.09 23.03,18.81 U3.8 | v21.56,1.71 28.69,1.58 31.49,4.23 U$1.16
  Bottom 0.254: v24.5,13.06 23.98,13.06 22.48,14.56 21.71,14.56 17.57,10.42 17.57,3.63 18.92,2.29 | v21.56,1.71 21.84,0.99 20.21,0.99 19.05,2.16 18.92,2.29 | I2C.1 18.92,2.29
SSEL1  (via drill 0.6)
  Top 0.254: U$2.23 11.06,12.89 v16.5,18.33 15.58,18.33 SPI.3 | v26.67,17.96 26.67,17.84 25.74,16.91 25.74,12.62 26.08,12.28 28.62,12.28 U$1.2
  Bottom 0.254: v16.5,18.33 19.93,18.33 20.55,17.71 26.41,17.71 v26.67,17.96
VBATT  (via drill 0.6)
  Top 0.254: 15.3,32.13 14.35,32.13 v13.81,31.59 | v25.7,26.79 24.88,26.79 C3.1 24.49,25.92 R3.2 25.03,25.87 26.62,24.27 | 26.62,24.27 R10.2 | 31.47,24.94 31.4,25.01 27.36,25.01 26.62,24.27 | 31.47,24.94 R5.2 32.44,26.48 C4.1 33.33,26.39 C15.1 34.27,23.6 C2.1 | 31.47,24.94 32.01,24.4 U4.3 32.57,24.08 33.4,23.24 33.4,22.35 32.18,22.35 U4.1
  Top 0.406: U1.3 1.91,29.8 0.91,30.81 0.91,33.35 2.05,34.49 8.08,34.49 | 8.08,34.49 9.41,33.16 9.41,31.61 9.37,31.57 9.37,31.53 8.73,30.88 6.84,30.88 JP2.2 | 15.75,34.28 L1.P$2 15.96,34.28 | 15.3,32.13 R4.2 | 8.08,34.49 9.2,35.61 14.63,35.61 15.75,34.48 15.75,34.28 | 15.75,34.28 15.75,33.99 14.68,32.91 14.68,32.09 R4.2 | R4.2 14.74,31.25 R6.2
  Bottom 0.254: v13.81,31.59 13.81,27.99 15.09,26.72 25.63,26.72 v25.7,26.79
VBUS
  Top 0.406: U1.4 1.45,26.09 C1.1 1.45,21.35 JP1.1
VIBE_PWM
  Top 0.254: U$3.+ 36.59,15.21 U$1.37
VIN
  Top 0.254: U2.5 16.55,31.92
  Top 0.406: 16.55,31.92 R4.1
XTALIN
  Top 0.254: Y1.3 23.29,3.41 | U$1.6 25.63,10.27 24.58,9.22 24.64,9.16 24.64,7.11 24.13,6.6 24.13,4.57 22.97,3.41 Y1.3 | Y1.3 21.21,3.41 C13.2
XTALOUT
  Top 0.254: C12.2 28.18,6.25 28.18,6.08 27.81,5.71 26.67,5.71 | 26.67,5.71 Y1.1 | 26.67,5.71 25.27,7.11 25.27,9.27 25.78,9.78 28.63,9.78 U$1.7

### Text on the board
tNames: Smart Watch Board V1 | 373 W13 | Designed by | Jonathan Meed | Joystick V1 | EECS 373 W2013 | David Jackson

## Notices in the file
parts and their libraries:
SparkFun-Connectors: Licensing: CC v3.0 Share-Alike You are welcome to use this library for commercial purposes.
